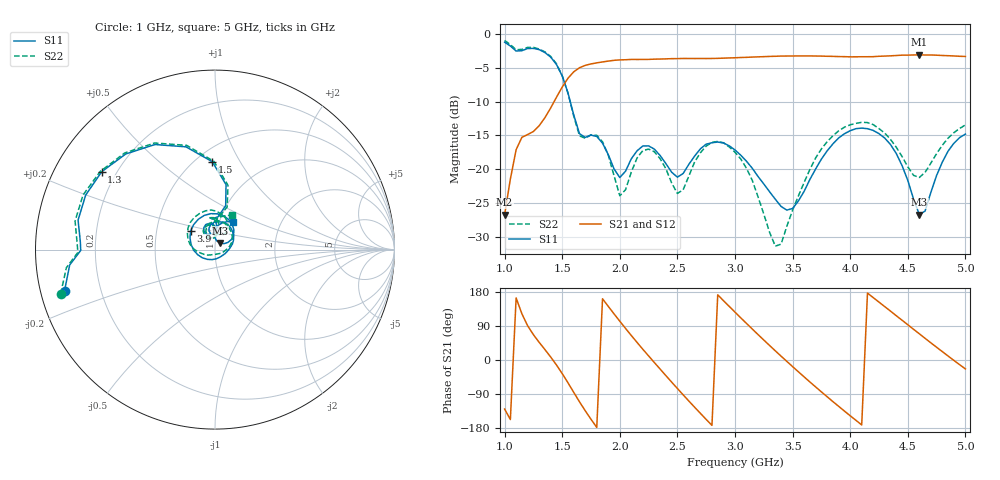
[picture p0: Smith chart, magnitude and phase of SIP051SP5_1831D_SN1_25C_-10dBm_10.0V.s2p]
# GHz  S  dB  R  50
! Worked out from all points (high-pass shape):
!   81 points, 1 GHz to 5 GHz, reference 50 ohm
!   highest |S21| = -3.08 dB at 4.6 GHz (marker M1); lowest = -26.7 dB at 1 GHz (marker M2)
!   |S21| within 3 dB of the highest: 1.574 GHz to end of sweep
!   lowest |S11| = -26.7 dB at 4.6 GHz (marker M3), VSWR 1.10, Z = 52.8 + j3.86 ohm
!   |S11| at or under -10 dB: 1.57 GHz to end of sweep
!   |S22| runs from -31.3 to -1.0 dB; largest |S21 - S12| = 0.0031
!   S11 on the Smith chart (normalised r, x): 1 GHz: 0.07, -0.13; 1.3 GHz: 0.15, +0.30; 1.5 GHz: 0.60, +0.77; 3.9 GHz: 0.75, +0.16; 5 GHz: 1.16, +0.36
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1  -1.22 -164.7  -26.71 -129.5  -26.65 -129.8  -0.96 -164.0
1.1  -2.52 -179.7  -17.10 163.7  -17.07 163.7  -2.34 -178.8
1.3  -2.31 145.5  -13.56 46.6  -13.58 46.8  -2.23 145.8
1.5  -6.20 91.8  -7.85 -35.8  -7.84 -35.7  -6.16 90.7
1.6  -11.96 76.3  -5.60 -85.3  -5.60 -85.5  -12.14 74.1
1.7  -15.29 96.1  -4.64 -134.0  -4.66 -134.0  -15.41 97.5
1.85  -16.13 88.4  -4.13 161.5  -4.13 161.7  -15.93 84.2
2.05  -20.26 118.9  -3.81 83.3  -3.81 83.2  -23.00 120.0
2.2  -16.55 110.0  -3.77 28.3  -3.77 28.4  -17.23 115.4
2.35  -17.96 88.3  -3.71 -24.0  -3.70 -24.0  -18.43 88.7
2.6  -19.24 107.9  -3.62 -108.5  -3.63 -108.4  -20.97 118.1
2.8  -16.07 81.7  -3.62 -172.5  -3.62 -172.5  -16.03 92.1
3  -17.14 44.2  -3.52 126.2  -3.50 126.3  -17.48 47.6
3.2  -21.05 9.7  -3.39 67.1  -3.38 67.2  -24.07 -1.1
3.4  -25.48 -38.0  -3.27 10.1  -3.27 10.2  -31.05 -105.1
3.7  -19.94 -163.8  -3.26 -71.1  -3.26 -71.0  -18.31 177.2
3.9  -15.36 142.6  -3.35 -122.3  -3.35 -122.4  -14.31 141.4
4.1  -13.91 96.5  -3.37 -171.3  -3.36 -171.4  -13.05 103.8
4.35  -16.34 46.5  -3.23 128.9  -3.23 128.9  -15.57 64.9
4.6  -26.68 51.8  -3.08 69.2  -3.09 69.1  -21.20 76.4
4.8  -18.92 89.2  -3.18 22.0  -3.18 21.9  -16.43 92.0
5  -14.80 56.5  -3.33 -23.6  -3.33 -23.6  -13.44 63.4
